VAR_GLOBAL CONSTANT
	cnMaxRecepeNum:				INT:=25;
END_VAR
VAR_GLOBAL
	vbtRecipeArr:				ARRAY[1..cnMaxRecepeNum] OF BOOL;
	strRecipeArr:				ARRAY[1..cnMaxRecepeNum] OF STRING;
	vbtFlash:					BOOL;
	vbtLoad:					BOOL;
	vbtSave:					BOOL;
	vbtDel:						BOOL;
	vbtLoadFromUSB:				BOOL;
	vbtSaveToUSB:				BOOL;
	ShowDiag: 					BOOL;
	DiagIndex:					INT;
	iSelectIndex:				INT;//当前选择的id号
	vbtYes: 					BOOL;
	vbtNo: 						BOOL;
	strShowDiagName:			STRING;
END_VAR
VAR_GLOBAL PERSISTENT
	strInputReceipeName AT%Q*:		STRING(30);
	strCurrentReceipeName AT%Q*:	STRING(30);
END_VAR
